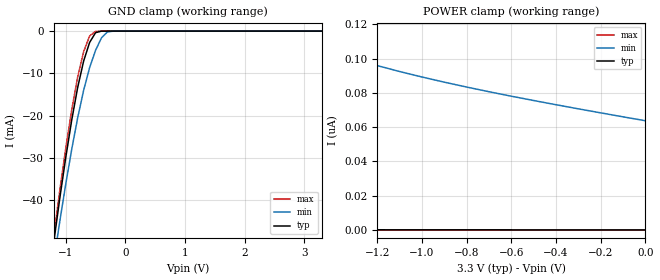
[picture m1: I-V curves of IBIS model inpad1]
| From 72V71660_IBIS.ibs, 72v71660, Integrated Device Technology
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|   Model inpad1
[Model]   inpad1
Model_type   Input
Polarity   Non-Inverting
Vinl =  0.80000V
Vinh =  2.00000V
C_comp   5.00000pF   NA   NA
[Temperature Range]   25.00000   100.00000   0.000
[Voltage Range]   3.30000V   3.00000V   3.60000V
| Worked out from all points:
|   GND clamp passes 1 mA (typ) near -0.53 V on its own axis
[GND_clamp]
| voltage   I(typ)   I(min)   I(max)
-3.3V     -310mA     -295.4mA   -315.4mA
-1.2V     -49.78mA   -54.27mA   -48.33mA
-1.1V     -39.5mA    -44.95mA   -37.65mA
-900mV    -21.04mA   -27.95mA   -18.63mA
-800mV    -13.32mA   -20.5mA    -10.85mA
-700mV    -7.09mA    -13.99mA   -4.876mA
-600mV    -2.698mA   -8.653mA   -1.161mA
-500mV    -374.6uA   -4.55mA    -53.22uA
-400mV    -11.83uA   -1.585mA   -1.231uA
-300mV    -285.2nA   -196.8uA   -25.38nA
-200mV    -6.527nA   -10.13uA   -459.3pA
3.3V      26.9pA     70.7nA     2.066pA
[POWER_clamp]
| voltage   I(typ)   I(min)   I(max)
-3.3V     3.879nA    456nA      684.6pA
-3V       2.36nA     327.1nA    413.6pA
-2.7V     1.415nA    242.1nA    246pA
-1.7V     242.2pA    118.8nA    39.53pA
-1.6V     203.7pA    113.3nA    32.78pA
-1.5V     171.8pA    108.3nA    27.21pA
-1.3V     123.7pA    99.68nA    18.83pA
-1.2V     105.8pA    95.94nA    15.74pA
-1V       78.71pA    89.29nA    11.07pA
-800mV    60.2pA     83.42nA    7.956pA
-600mV    47.4pA     78.08nA    5.874pA
0V        26.91pA    63.75nA    2.762pA
